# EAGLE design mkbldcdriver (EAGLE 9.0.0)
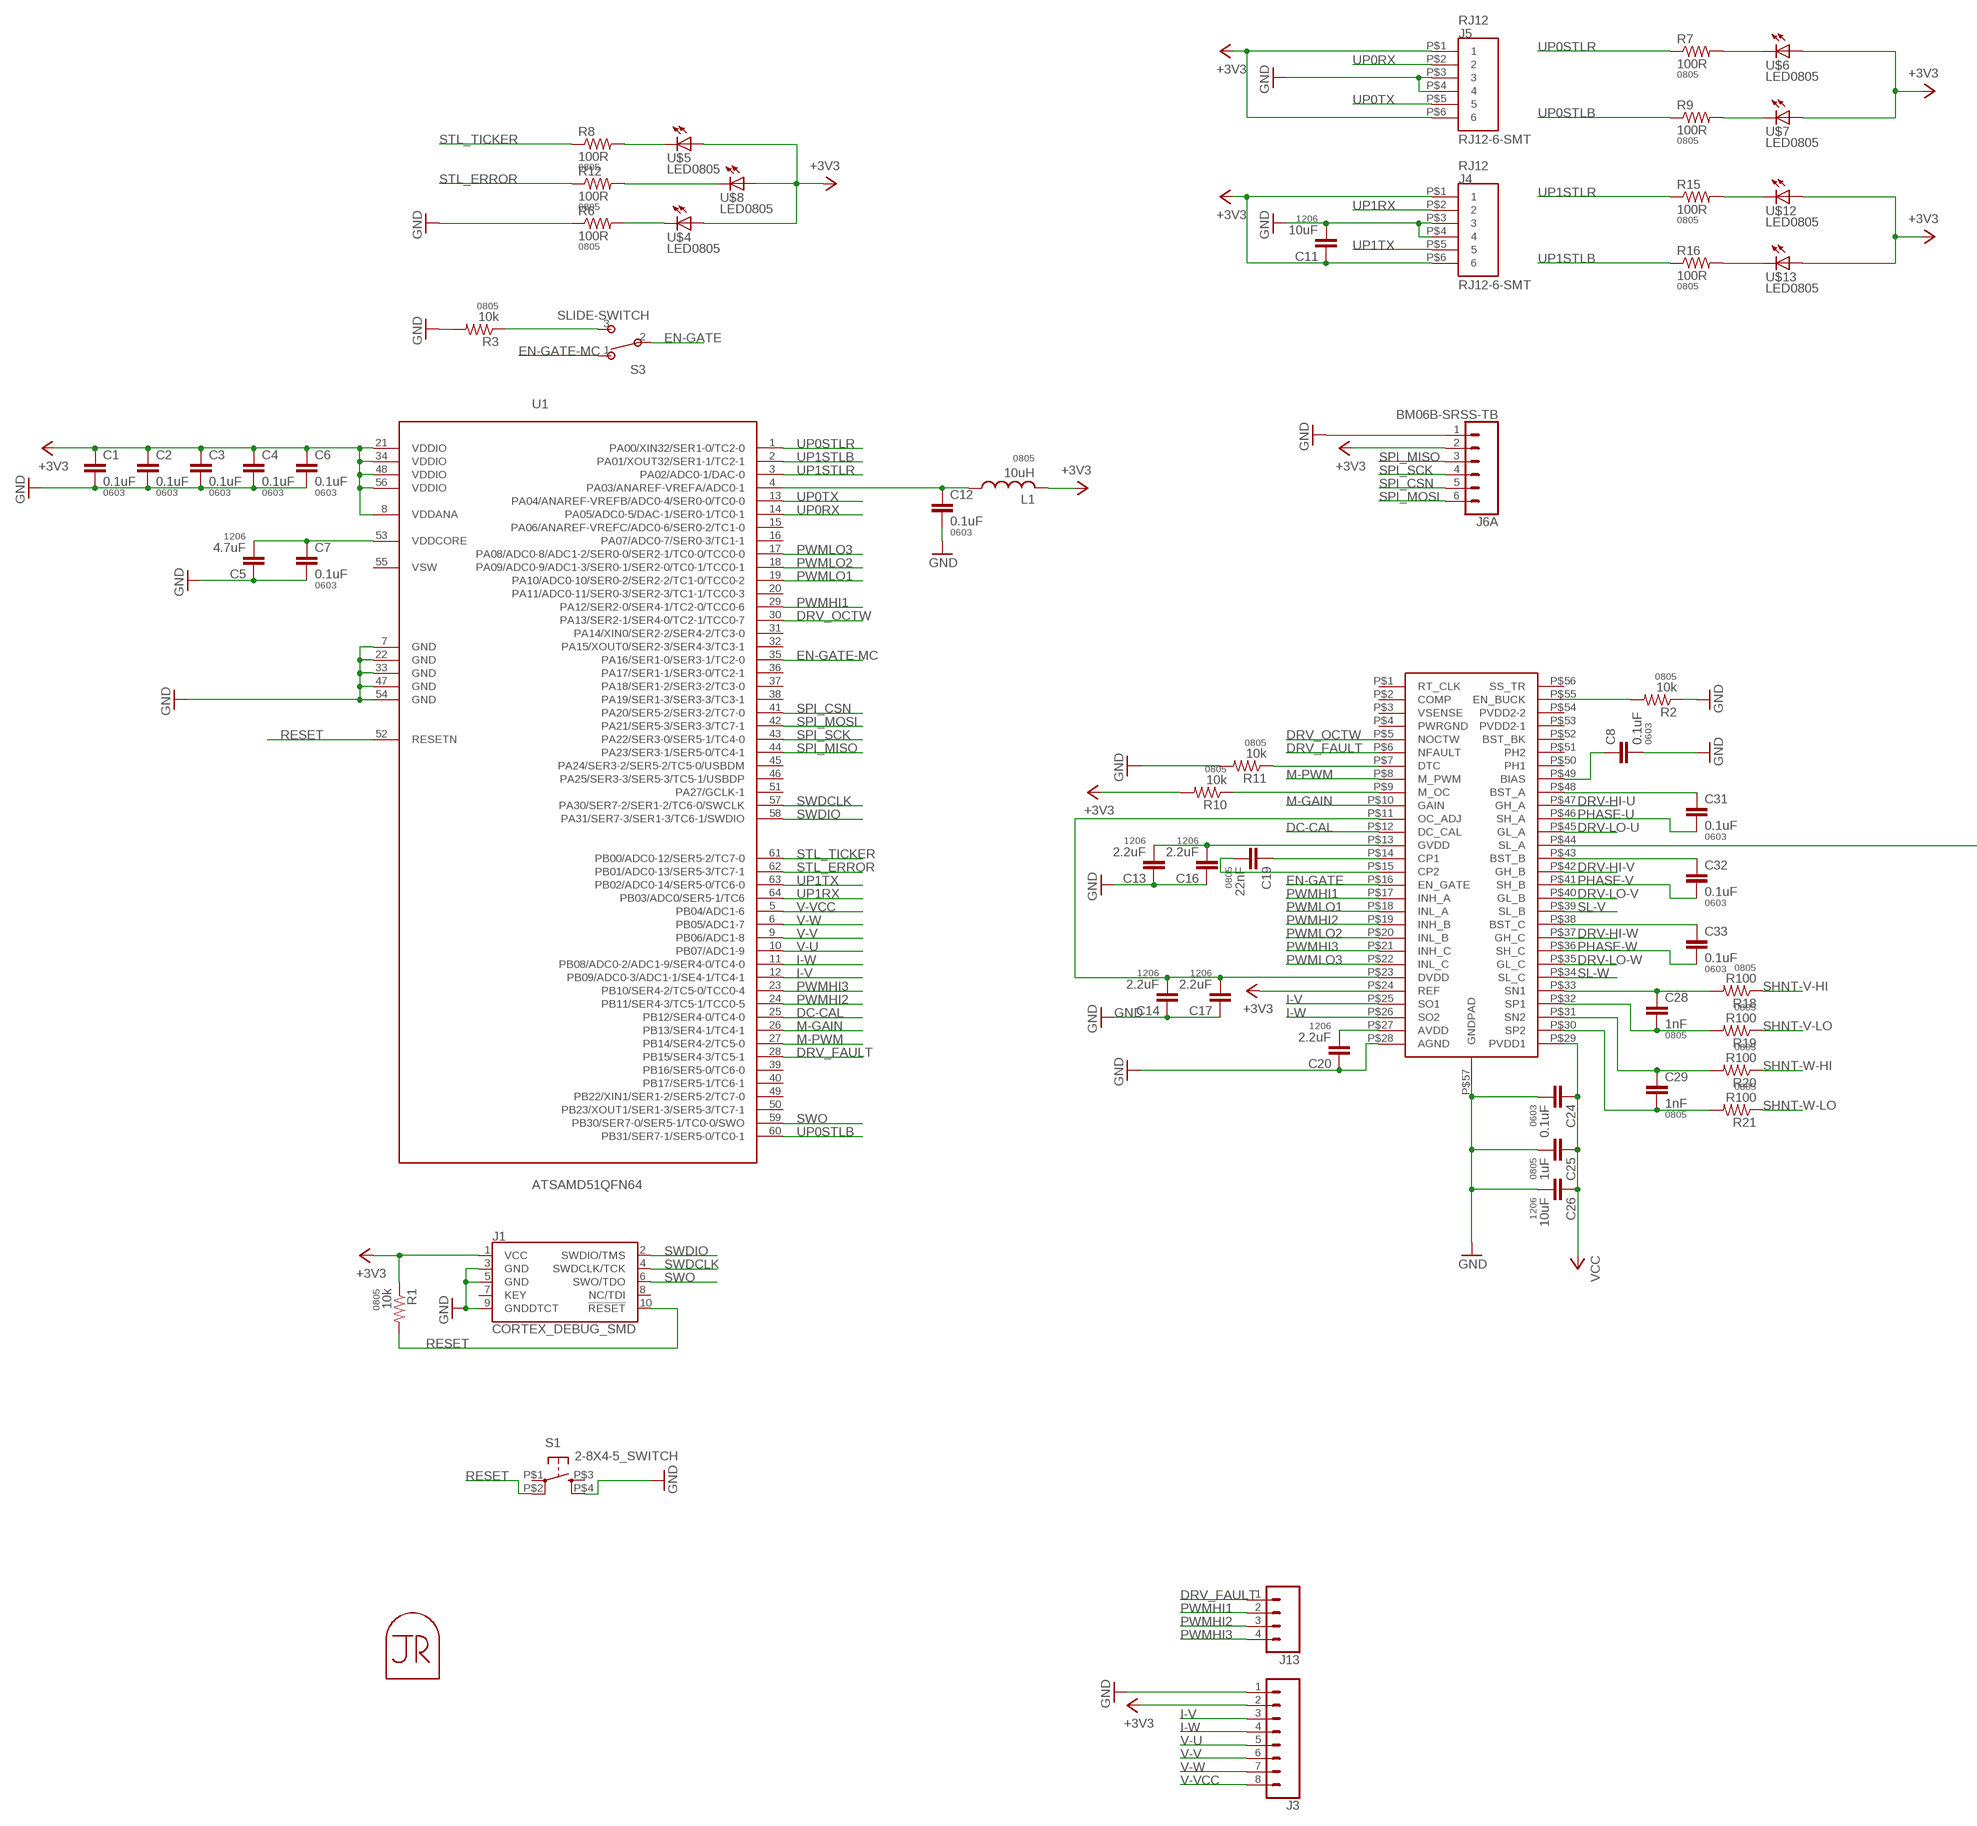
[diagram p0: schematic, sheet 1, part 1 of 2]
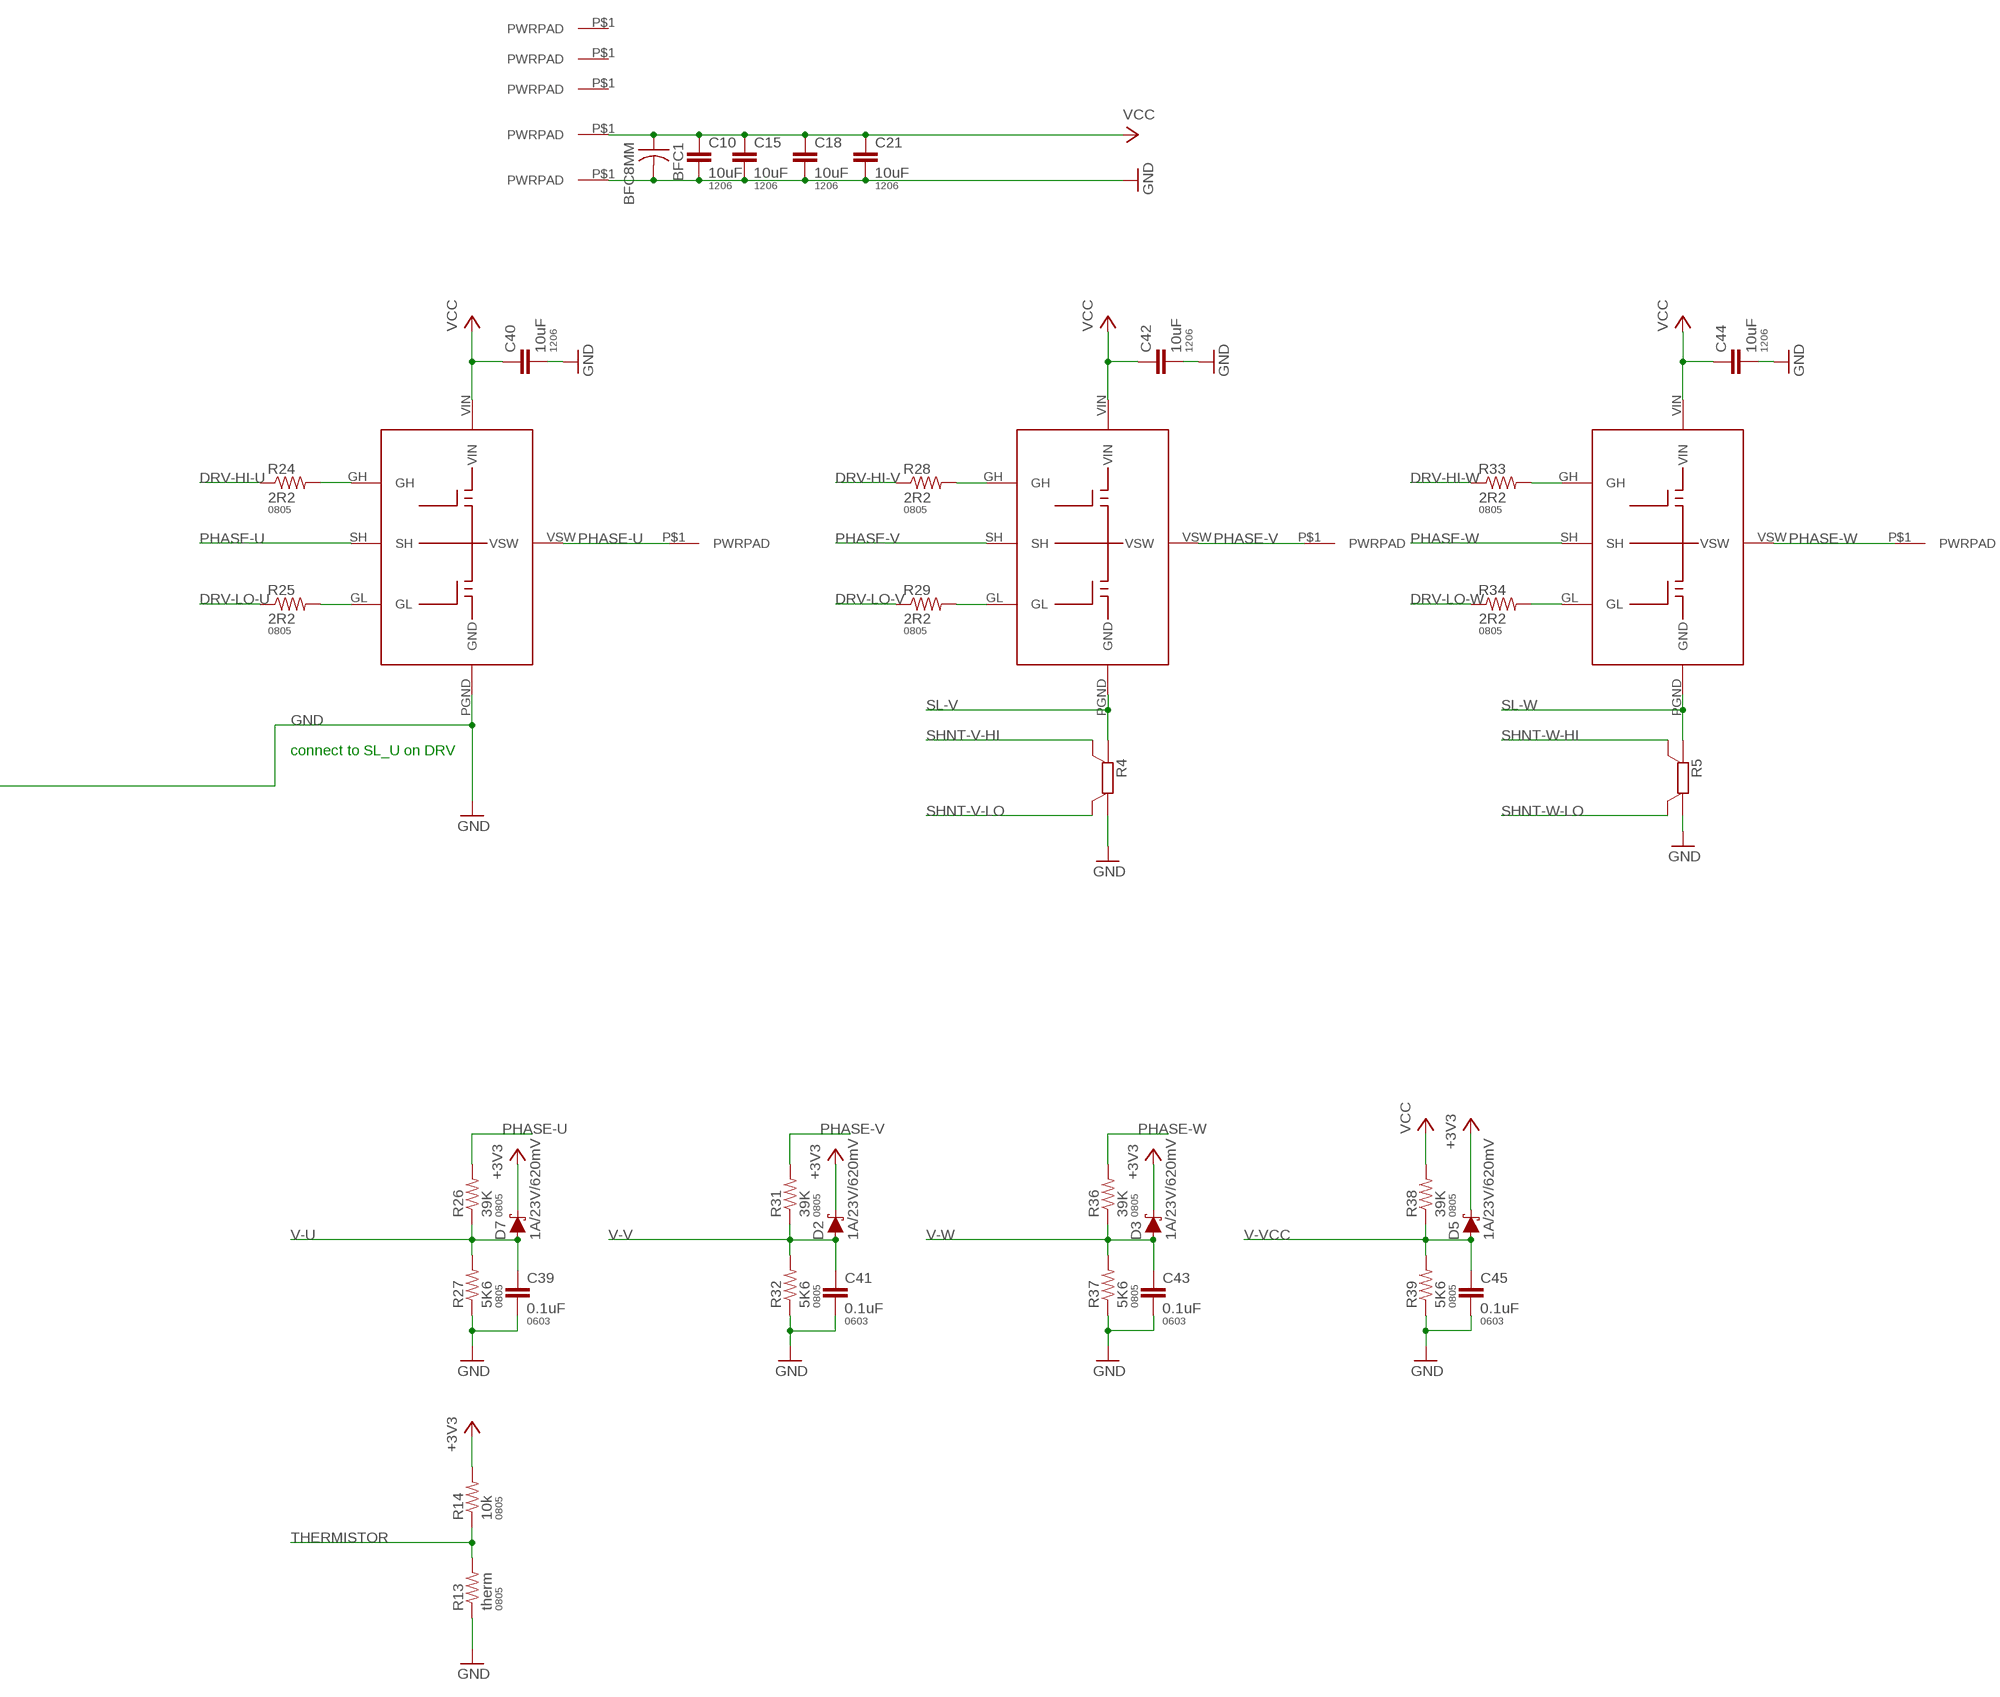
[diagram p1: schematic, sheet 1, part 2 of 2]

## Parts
BFC1  BFC8MM  [BFC-8MM]
C1  0.1uF  CAP0603-CAP  [0603-CAP]
C2  0.1uF  CAP0603-CAP  [0603-CAP]
C3  0.1uF  CAP0603-CAP  [0603-CAP]
C4  0.1uF  CAP0603-CAP  [0603-CAP]
C5  4.7uF  CAP1206  [1206]
C6  0.1uF  CAP0603-CAP  [0603-CAP]
C7  0.1uF  CAP0603-CAP  [0603-CAP]
C8  0.1uF  CAP0603-CAP  [0603-CAP]
C10  10uF  CAP1206  [1206]
C11  10uF  CAP1206  [1206]
C12  0.1uF  CAP0603-CAP  [0603-CAP]
C13  2.2uF  CAP1206  [1206]
C14  2.2uF  CAP1206  [1206]
C15  10uF  CAP1206  [1206]
C16  2.2uF  CAP1206  [1206]
C17  2.2uF  CAP1206  [1206]
C18  10uF  CAP1206  [1206]
C19  22nF  CAP0805  [0805]
C20  2.2uF  CAP1206  [1206]
C21  10uF  CAP1206  [1206]
C24  0.1uF  CAP0603-CAP  [0603-CAP]
C25  1uF  CAP0805  [0805]
C26  10uF  CAP1206  [1206]
C28  1nF  CAP0805  [0805]
C29  1nF  CAP0805  [0805]
C31  0.1uF  CAP0603-CAP  [0603-CAP]
C32  0.1uF  CAP0603-CAP  [0603-CAP]
C33  0.1uF  CAP0603-CAP  [0603-CAP]
C39  0.1uF  CAP0603-CAP  [0603-CAP]
C40  10uF  CAP1206  [1206]
C41  0.1uF  CAP0603-CAP  [0603-CAP]
C42  10uF  CAP1206  [1206]
C43  0.1uF  CAP0603-CAP  [0603-CAP]
C44  10uF  CAP1206  [1206]
C45  0.1uF  CAP0603-CAP  [0603-CAP]
D2  1A/23V/620mV  DIODE-SCHOTTKY-BAT20J  [SOD-323]
D3  1A/23V/620mV  DIODE-SCHOTTKY-BAT20J  [SOD-323]
D5  1A/23V/620mV  DIODE-SCHOTTKY-BAT20J  [SOD-323]
D7  1A/23V/620mV  DIODE-SCHOTTKY-BAT20J  [SOD-323]
J1  CORTEX_DEBUG_SMD  [SAMTECH_FTSH-105-01]
J3  CONN_08NO_SILK_FEMALE_PTH  [1X08_NO_SILK]
J4  RJ12-6-SMT  [RJ12-6-SMT]
J5  RJ12-6-SMT  [RJ12-6-SMT]
J6  BM06B-SRSS-TB  JST_6_PIN_HORIZONTAL  [JST-6-SMD-HORI-1.0MM]
J7  PWRPAD  [PWRPAD_M3-PEM-MOUNT]
J8  PWRPAD  [PWRPAD_M3-PEM-MOUNT]
J9  PWRPAD  [PWRPAD_M3-PEM-MOUNT]
J10  PWRPAD  [PWRPAD_M3-PEM-MOUNT]
J11  PWRPAD  [PWRPAD_M3-PEM-MOUNT]
J12  PWRPADM3  [PWRPAD_3-25MM]
J13  CONN_041X04_NO_SILK  [1X04_NO_SILK]
J14  PWRPADM3  [PWRPAD_3-25MM]
J15  PWRPADM3  [PWRPAD_3-25MM]
L1  10uH  INDUCTOR-0805  [0805]
R1  10k  RESISTOR0805-RES  [0805]
R2  10k  RESISTOR0805-RES  [0805]
R3  10k  RESISTOR0805-RES  [0805]
R4  R_SHUNT2512  [R2512]
R5  R_SHUNT2512  [R2512]
R6  100R  RESISTOR0805-RES  [0805]
R7  100R  RESISTOR0805-RES  [0805]
R8  100R  RESISTOR0805-RES  [0805]
R9  100R  RESISTOR0805-RES  [0805]
R10  10k  RESISTOR0805-RES  [0805]
R11  10k  RESISTOR0805-RES  [0805]
R12  100R  RESISTOR0805-RES  [0805]
R13  therm  RESISTOR0805-RES  [0805]
R14  10k  RESISTOR0805-RES  [0805]
R15  100R  RESISTOR0805-RES  [0805]
R16  100R  RESISTOR0805-RES  [0805]
R18  R100  RESISTOR0805-RES  [0805]
R19  R100  RESISTOR0805-RES  [0805]
R20  R100  RESISTOR0805-RES  [0805]
R21  R100  RESISTOR0805-RES  [0805]
R24  2R2  RESISTOR0805-RES  [0805]
R25  2R2  RESISTOR0805-RES  [0805]
R26  39K  RESISTOR0805-RES  [0805]
R27  5K6  RESISTOR0805-RES  [0805]
R28  2R2  RESISTOR0805-RES  [0805]
R29  2R2  RESISTOR0805-RES  [0805]
R31  39K  RESISTOR0805-RES  [0805]
R32  5K6  RESISTOR0805-RES  [0805]
R33  2R2  RESISTOR0805-RES  [0805]
R34  2R2  RESISTOR0805-RES  [0805]
R36  39K  RESISTOR0805-RES  [0805]
R37  5K6  RESISTOR0805-RES  [0805]
R38  39K  RESISTOR0805-RES  [0805]
R39  5K6  RESISTOR0805-RES  [0805]
S1  2-8X4-5_SWITCH  [TACT-SWITCH-KMR6]
S3  SLIDE-SWITCH  [AYZ0102AGRLC]
U1  ATSAMD51QFN64  [QFN-64-9X9MM]
U2  DRV8302  [HTSSOP-56]
U$4  LED0805  [LED0805]
U$5  LED0805  [LED0805]
U$6  LED0805  [LED0805]
U$7  LED0805  [LED0805]
U$8  LED0805  [LED0805]
U$9  INTEGRATED_HALF-CSD88599SON  [SON-5X6]
U$10  INTEGRATED_HALF-CSD88599SON  [SON-5X6]
U$11  INTEGRATED_HALF-CSD88599SON  [SON-5X6]
U$12  LED0805  [LED0805]
U$13  LED0805  [LED0805]
U$14  JRTOMBSTONE  [JRTOMBSTONE]

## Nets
+3V3: C1.1 C2.1 C3.1 C4.1 C6.1 C11.1 D2.C D3.C D5.C D7.C J1.1(VCC) J3.2 J4.P$1 J4.P$6 J5.P$1 J5.P$6 J6.2 L1.2 R1.1 R10.2 R14.2 U1.8(VDDANA) U1.21(VDDIO) U1.34(VDDIO) U1.48(VDDIO) U1.56(VDDIO) U2.P$24(REF) U$4.1(A) U$5.1(A) U$6.1(A) U$7.1(A) U$8.1(A) U$12.1(A) U$13.1(A)
CP1: C19.1 U2.P$14(CP1)
CP2: C19.2 U2.P$15(CP2)
DC-CAL: U1.25(PB12/SER4-0/TC4-0) U2.P$12(DC_CAL)
DRV-HI-U: R24.1 U2.P$47(GH_A)
DRV-HI-V: R28.1 U2.P$42(GH_B)
DRV-HI-W: R33.1 U2.P$37(GH_C)
DRV-LO-U: R25.1 U2.P$45(GL_A)
DRV-LO-V: R29.1 U2.P$40(GL_B)
DRV-LO-W: R34.1 U2.P$35(GL_C)
DRV_FAULT: J13.1 U1.28(PB15/SER4-3/TC5-1) U2.P$6(NFAULT)
DRV_OCTW: U1.30(PA13/SER2-1/SER4-0/TC2-1/TCC0-7) U2.P$5(NOCTW)
EN-GATE: S3.2 U2.P$16(EN_GATE)
EN-GATE-MC: S3.1 U1.35(PA16/SER1-0/SER3-1/TC2-0)
GND: BFC1.P$2 C1.2 C2.2 C3.2 C4.2 C5.1 C6.2 C7.2 C8.2 C10.2 C11.2 C12.2 C13.1 C14.1 C15.2 C16.1 C17.1 C18.2 C20.1 C21.2 C24.2 C25.2 C26.2 C39.2 C40.2 C41.2 C42.2 C43.2 C44.2 C45.2 J1.3(GND) J1.5(GND) J1.9(GNDDTCT) J3.1 J4.P$3 J4.P$4 J5.P$3 J5.P$4 J6.1 J9.P$1(PWRPAD) R2.1 R3.2 R4.A R5.A R6.1 R11.2 R13.1 R27.1 R32.1 R37.1 R39.1 S1.P$4(S1) U1.7(GND) U1.22(GND) U1.33(GND) U1.47(GND) U1.54(GND) U2.P$28(AGND) U2.P$44(SL_A) U2.P$57(GNDPAD) U$9.PGND(GND)
I-V: J3.3 U1.12(PB09/ADC0-3/ADC1-1/SE4-1/TC4-1) U2.P$25(SO1)
I-W: J3.4 U1.11(PB08/ADC0-2/ADC1-9/SER4-0/TC4-0) U2.P$26(SO2)
M-GAIN: U1.26(PB13/SER4-1/TC4-1) U2.P$10(GAIN)
M-PWM: U1.27(PB14/SER4-2/TC5-0) U2.P$8(M_PWM)
N$1: R7.2 U$6.2(C)
N$2: R25.2 U$9.GL
N$3: R24.2 U$9.GH
N$4: R28.2 U$10.GH
N$5: R33.2 U$11.GH
N$6: R34.2 U$11.GL
N$7: C33.1 U2.P$38(BST_C)
N$8: C32.1 U2.P$43(BST_B)
N$9: C31.1 U2.P$48(BST_A)
N$10: R2.2 U2.P$55(EN_BUCK)
N$11: C20.2 U2.P$27(AVDD)
N$13: C28.1 R18.2 U2.P$33(SN1)
N$14: C28.2 R19.2 U2.P$32(SP1)
N$15: C29.1 R20.2 U2.P$31(SN2)
N$16: C29.2 R21.2 U2.P$30(SP2)
N$18: C13.2 C16.2 U2.P$13(GVDD)
N$19: C8.1 U2.P$49(BIAS)
N$20: C14.2 C17.2 U2.P$11(OC_ADJ) U2.P$23(DVDD)
N$21: R11.1 U2.P$7(DTC)
N$22: R9.2 U$7.2(C)
N$23: R12.2 U$8.2(C)
N$24: R29.2 U$10.GL
N$25: R10.1 U2.P$9(M_OC)
N$26: R3.1 S3.3
N$27: R15.2 U$12.2(C)
N$28: R16.2 U$13.2(C)
N$34: C12.1 L1.1 U1.4(PA03/ANAREF-VREFA/ADC0-1)
N$35: R6.2 U$4.2(C)
N$36: R8.2 U$5.2(C)
PHASE-U: C31.2 J7.P$1(PWRPAD) R26.2 U2.P$46(SH_A) U$9.SH U$9.VSW
PHASE-V: C32.2 J10.P$1(PWRPAD) R31.2 U2.P$41(SH_B) U$10.SH U$10.VSW
PHASE-W: C33.2 J11.P$1(PWRPAD) R36.2 U2.P$36(SH_C) U$11.SH U$11.VSW
PWMHI1: J13.2 U1.29(PA12/SER2-0/SER4-1/TC2-0/TCC0-6) U2.P$17(INH_A)
PWMHI2: J13.3 U1.24(PB11/SER4-3/TC5-1/TCC0-5) U2.P$19(INH_B)
PWMHI3: J13.4 U1.23(PB10/SER4-2/TC5-0/TCC0-4) U2.P$21(INH_C)
PWMLO1: U1.19(PA10/ADC0-10/SER0-2/SER2-2/TC1-0/TCC0-2) U2.P$18(INL_A)
PWMLO2: U1.18(PA09/ADC0-9/ADC1-3/SER0-1/SER2-0/TC0-1/TCC0-1) U2.P$20(INL_B)
PWMLO3: U1.17(PA08/ADC0-8/ADC1-2/SER0-0/SER2-1/TC0-0/TCC0-0) U2.P$22(INL_C)
RESET: J1.10(!RESET) R1.2 S1.P$2(P1) U1.52(RESETN)
SHNT-V-HI: R4.SB R18.1
SHNT-V-LO: R4.SA R19.1
SHNT-W-HI: R5.SB R20.1
SHNT-W-LO: R5.SA R21.1
SL-V: R4.B U2.P$39(SL_B) U$10.PGND(GND)
SL-W: R5.B U2.P$34(SL_C) U$11.PGND(GND)
SPI_CSN: J6.5 U1.41(PA20/SER5-2/SER3-2/TC7-0)
SPI_MISO: J6.3 U1.44(PA23/SER3-1/SER5-0/TC4-1)
SPI_MOSI: J6.6 U1.42(PA21/SER5-3/SER3-3/TC7-1)
SPI_SCK: J6.4 U1.43(PA22/SER3-0/SER5-1/TC4-0)
STL_ERROR: R12.1 U1.62(PB01/ADC0-13/SER5-3/TC7-1)
STL_TICKER: R8.1 U1.61(PB00/ADC0-12/SER5-2/TC7-0)
SWDCLK: J1.4(SWDCLK/TCK) U1.57(PA30/SER7-2/SER1-2/TC6-0/SWCLK)
SWDIO: J1.2(SWDIO/TMS) U1.58(PA31/SER7-3/SER1-3/TC6-1/SWDIO)
SWO: J1.6(SWO/TDO) U1.59(PB30/SER7-0/SER5-1/TC0-0/SWO)
THERMISTOR: R13.2 R14.1
UP0RX: J5.P$2 U1.14(PA05/ADC0-5/DAC-1/SER0-1/TC0-1)
UP0STLB: R9.1 U1.60(PB31/SER7-1/SER5-0/TC0-1)
UP0STLR: R7.1 U1.1(PA00/XIN32/SER1-0/TC2-0)
UP0TX: J5.P$5 U1.13(PA04/ANAREF-VREFB/ADC0-4/SER0-0/TC0-0)
UP1RX: J4.P$2 U1.64(PB03/ADC0/SER5-1/TC6)
UP1STLB: R16.1 U1.2(PA01/XOUT32/SER1-1/TC2-1)
UP1STLR: R15.1 U1.3(PA02/ADC0-1/DAC-0)
UP1TX: J4.P$5 U1.63(PB02/ADC0-14/SER5-0/TC6-0)
V-U: C39.1 D7.A J3.5 R26.1 R27.2 U1.10(PB07/ADC1-9)
V-V: C41.1 D2.A J3.6 R31.1 R32.2 U1.9(PB06/ADC1-8)
V-VCC: C45.1 D5.A J3.8 R38.1 R39.2 U1.5(PB04/ADC1-6)
V-W: C43.1 D3.A J3.7 R36.1 R37.2 U1.6(PB05/ADC1-7)
VCC: BFC1.P$1 C10.1 C15.1 C18.1 C21.1 C24.1 C25.1 C26.1 C40.1 C42.1 C44.1 J8.P$1(PWRPAD) R38.2 U2.P$29(PVDD1) U$9.VIN U$10.VIN U$11.VIN
VDDCORE: C5.2 C7.1 U1.53(VDDCORE)
Unconnected: J1.7(KEY) J1.8(NC/TDI) J6.M1 J6.M2 J12.P$1(PWRPAD) J14.P$1(PWRPAD) J15.P$1(PWRPAD) S1.P$1(P) S1.P$3(S) U1.15(PA06/ANAREF-VREFC/ADC0-6/SER0-2/TC1-0) U1.16(PA07/ADC0-7/SER0-3/TC1-1) U1.20(PA11/ADC0-11/SER0-3/SER2-3/TC1-1/TCC0-3) U1.31(PA14/XIN0/SER2-2/SER4-2/TC3-0) U1.32(PA15/XOUT0/SER2-3/SER4-3/TC3-1) U1.36(PA17/SER1-1/SER3-0/TC2-1) U1.37(PA18/SER1-2/SER3-2/TC3-0) U1.38(PA19/SER1-3/SER3-3/TC3-1) U1.39(PB16/SER5-0/TC6-0) U1.40(PB17/SER5-1/TC6-1) U1.45(PA24/SER3-2/SER5-2/TC5-0/USBDM) U1.46(PA25/SER3-3/SER5-3/TC5-1/USBDP) U1.49(PB22/XIN1/SER1-2/SER5-2/TC7-0) U1.50(PB23/XOUT1/SER1-3/SER5-3/TC7-1) U1.51(PA27/GCLK-1) U1.55(VSW) U2.P$1(RT_CLK) U2.P$2(COMP) U2.P$3(VSENSE) U2.P$4(PWRGND) U2.P$50(PH1) U2.P$51(PH2) U2.P$52(BST_BK) U2.P$53(PVDD2-1) U2.P$54(PVDD2-2) U2.P$56(SS_TR)

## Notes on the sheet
- connect to SL_U on DRV

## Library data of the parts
BFC1 = power:BFC
C1-C4 C6-C8 C12 C24 C31-C33 C39 C41 C43 C45 = borkedlabs-passives:CAP: Capacitor; PACKAGE: 0603
C5 C10 C11 C13-C18 C20 C21 C26 C40 C42 C44 = borkedlabs-passives:CAP: Capacitor; PACKAGE: 1206
C19 C25 C28 C29 = borkedlabs-passives:CAP: Capacitor; PACKAGE: 0805
D2 D3 D5 D7 = SparkFun-DiscreteSemi:DIODE-SCHOTTKY: Schottky diode; PROD_ID: DIO-11623
J1 = SparkFun-Connectors:CORTEX_DEBUG: Cortex Debug Connector - 10 pin Supports JTAG debug, Serial Wire debug, and Serial Wire Viewer. PTH and SMD connector options available. General Connector Information Products: PTH Connector -via Digi-Key SparkFun PSoc SparkFun T
J3 = SparkFun-Connectors:CONN_08: Multi connection point. Often used as Generic Header-pin footprint for 0.1 inch spaced/style header connections On any of the 0.1 inch spaced packages, you can populate with these: Break Away Headers - Straight (PRT-00116) Break Away Male Headers - Right Angle (PRT-00553) Female Headers (PRT-00115)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; PROD_ID: CONN-08438
J4 J5 = connector:RJ12-6-SMT
J6 = SparkFun-Connectors:JST_6_PIN_HORIZONTAL: JST 6 pin horizontal connector JST-SH type. Here is the connector we sell at SparkFun: name (XXX-00000) Datasheet It was used on these SparkFun products: name (XXX-00000) name (XXX-00000); PROD_ID: XXX-00000
J7-J12 J14 J15 = power:PWRPAD
J13 = SparkFun-Connectors:CONN_04: Multi connection point. Often used as Generic Header-pin footprint for 0.1 inch spaced/style header connections On any of the 0.1 inch spaced packages, you can populate with these: Break Away Headers - Straight (PRT-00116) Break Away Male Headers - Right Angle (PRT-00553) Female Headers (PRT-00115)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; PROD_ID: CONN-09696
L1 = borkedlabs-passives:INDUCTOR; PACKAGE: 0805
R1-R3 R6-R16 R18-R21 R24-R29 R31-R34 R36-R39 = borkedlabs-passives:RESISTOR: Resistor; PACKAGE: 0805
R4 R5 = power:R_SHUNT: Resistor Basic schematic elements and footprints for 0603, 1206, and PTH resistors.
S1 = fab:2-8X4-5_SWITCH
S3 = fab:SLIDE-SWITCH: SMD slide-switch AYZ0102AGRLC as found in the fablab inventory. Includes the mounting holes. Made by Zaerc.
U1 = atsam:ATSAMD51
U2 = power:DRV8302
U$4-U$8 U$12 U$13 = lights:LED: LED
U$9-U$11 = power:INTEGRATED_HALF-CSD88599
U$14 = connector:JRTOMBSTONE

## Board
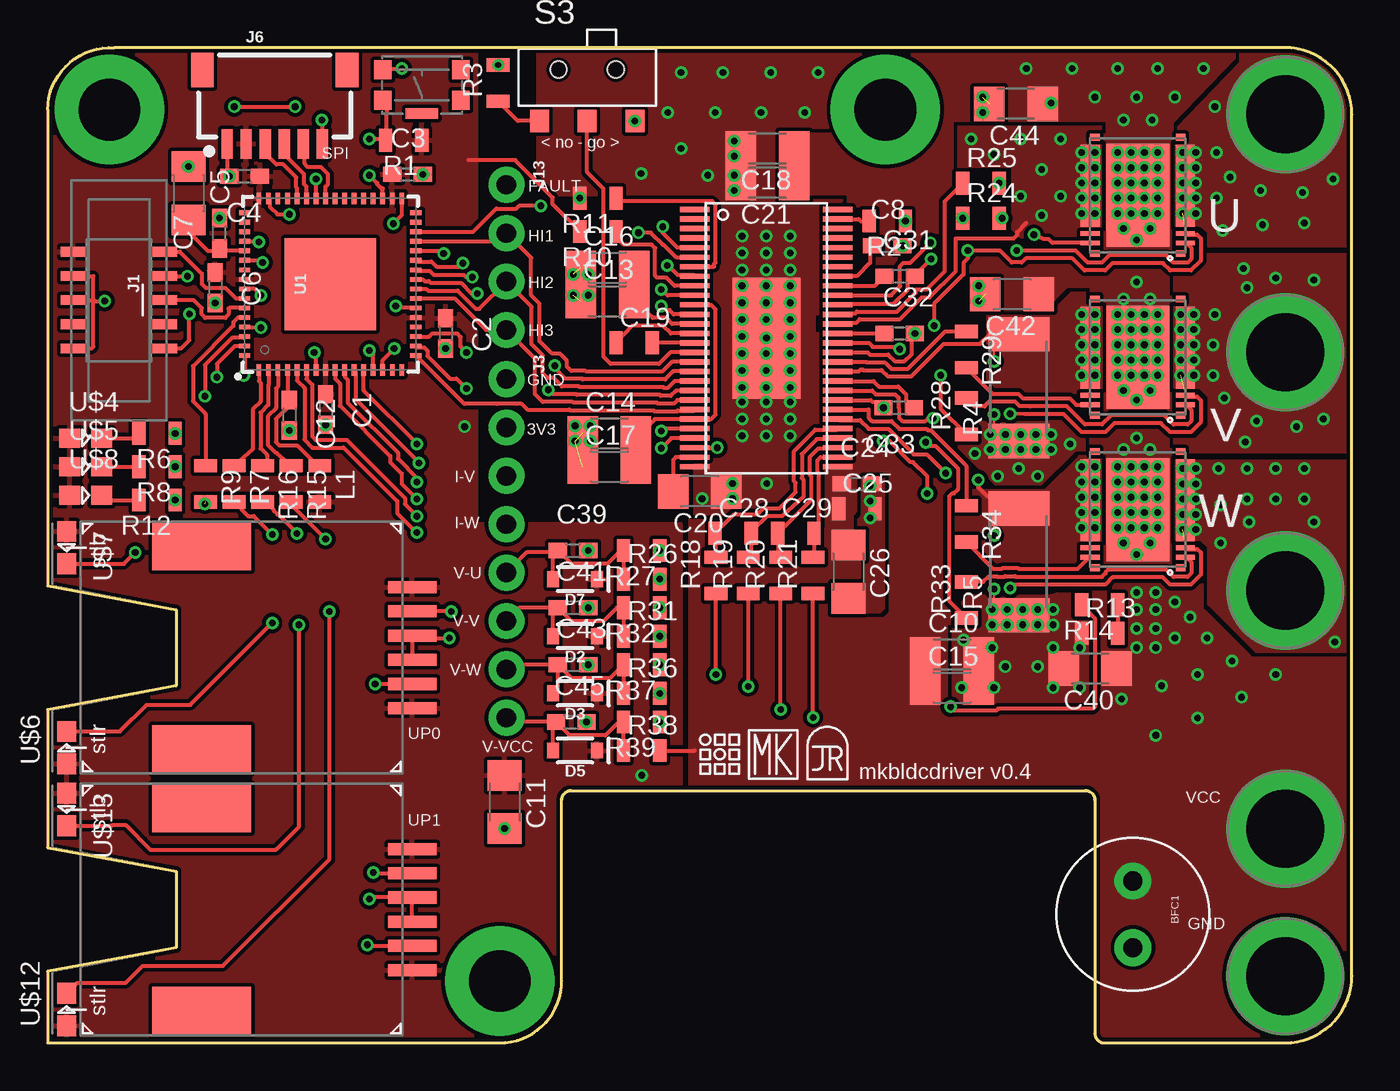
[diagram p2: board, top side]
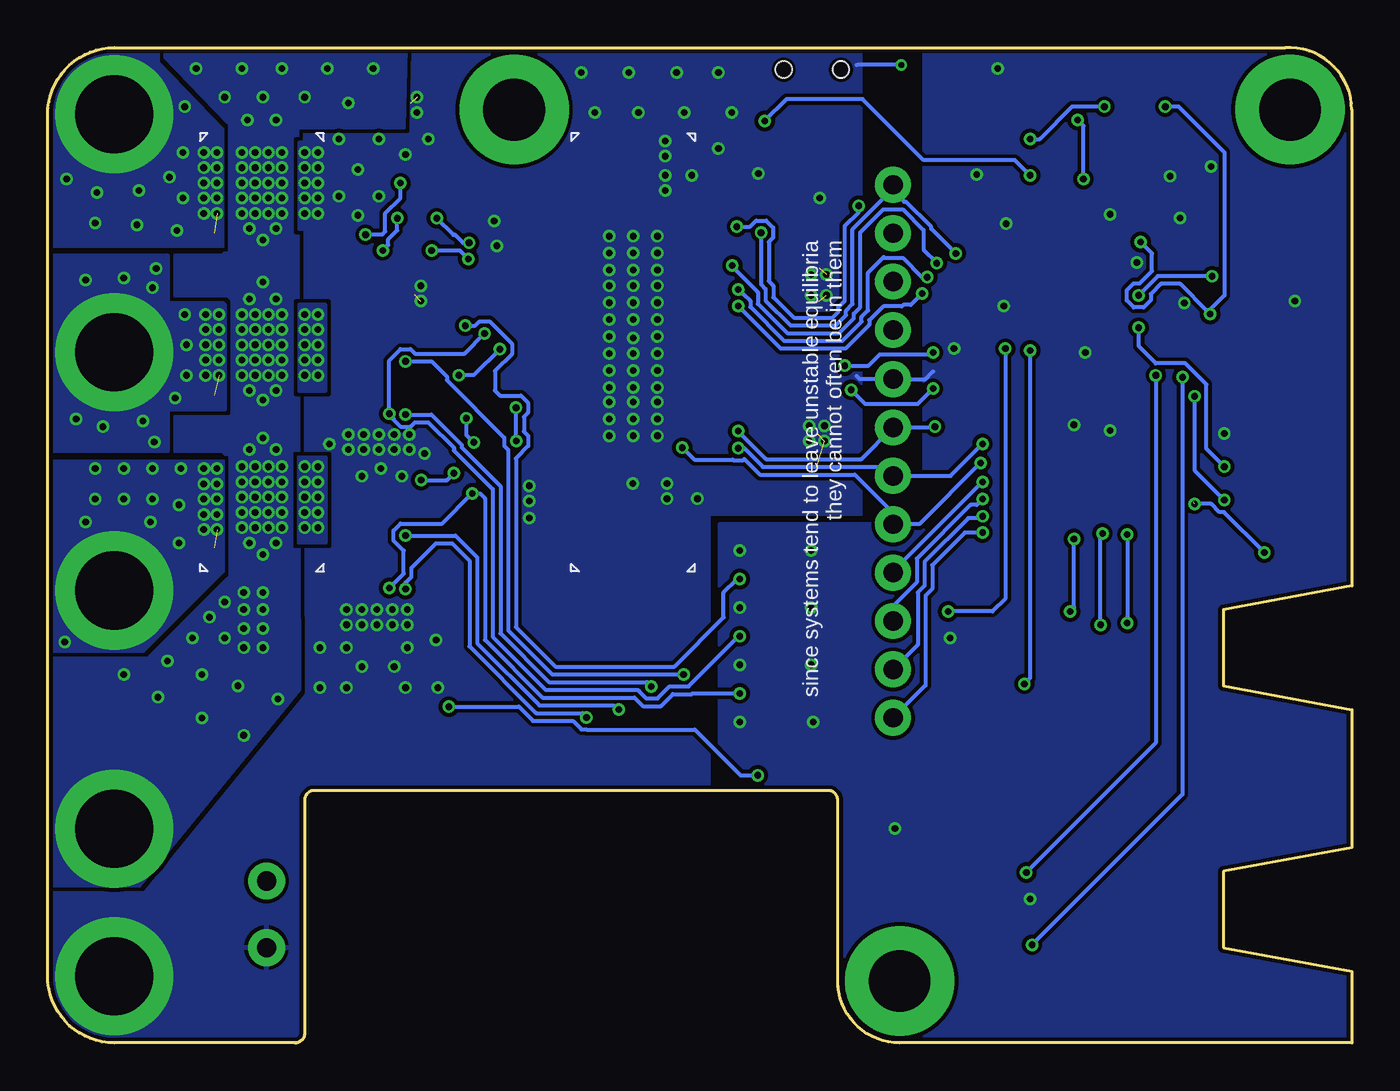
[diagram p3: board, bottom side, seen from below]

Size 68.5 x 52.25 mm. Coordinates in mm from the lower left corner, seen from the top.
Outline: 0,49 arc-92 3.5,52.25 65,52.25 arc-90 68.5,48.75 68.5,3.5 arc-90 65,0 55.5,0 arc-90 55,0.5 55,12.75 arc90 54.5,13.25 27.5,13.25 arc90 27,12.75 27,3.25 arc-90 23.75,0 0,0 0,3.75 6.75,5 6.75,9 0,10.25 0,17.5 6.75,18.75 6.75,22.75 0,24 0,49
Copper layers (1*16): Top 0.035mm / dielectric 1.5mm / Bottom 0.035mm
Design rules "default *": minimum track width 8mil, minimum drill 0.35mm, track to track 8mil, track to pad 8mil, pad to pad 8mil, via to via 8mil, smd to smd 8mil, copper to edge 8mil, drill to drill 8mil, minimum pad ring 10mil, minimum via ring 6mil, stop-mask expansion 4mil, vias tented up to drill 20mil, thermal gap 8mil

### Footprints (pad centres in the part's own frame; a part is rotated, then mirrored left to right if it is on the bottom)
BFC-8MM = drill 1 pad 1.93: P$1 -1.75,0; P$2 1.75,0
0603-CAP = smd 0.96 x 0.8: 1 -0.8,0; 2 0.8,0
1206 = smd 1.6 x 1.8: 1 -1.4,0; 2 1.4,0
0805 = smd 0.7 x 1.2: 1 -0.95,0; 2 0.95,0
SOD-323 = smd 0.63 x 0.83: A 1.15,0; C -1.15,0
SAMTECH_FTSH-105-01 = smd 0.508 x 1.27: 1 -2.54,-2.413; 2 -2.54,2.413; 3 -1.27,-2.413; 4 -1.27,2.413; 5 0,-2.413; 6 0,2.413; 7 1.27,-2.413; 8 1.27,2.413; 9 2.54,-2.413; 10 2.54,2.413
1X08_NO_SILK = drill 1.016 pad 1.88: 1 0,0; 2 2.54,0; 3 5.08,0; 4 7.62,0; 5 10.16,0; 6 12.7,0; 7 15.24,0; 8 17.78,0
RJ12-6-SMT = smd 0.635 x 2.54: P$1 -3.175,17.399; P$2 -1.905,17.399; P$3 -0.635,17.399; P$4 0.635,17.399; P$5 1.905,17.399; P$6 3.175,17.399 | smd 2.54 x 5.207: P$7 -5.334,6.35; P$8 5.334,6.35
JST-6-SMD-HORI-1.0MM = smd 0.6 x 1.55: 1 -2.5,-4.775; 2 -1.5,-4.775; 3 -0.5,-4.775; 4 0.5,-4.775; 5 1.5,-4.775; 6 2.5,-4.775 | smd 1.2 x 1.8: M1 -3.8,-0.9; M2 3.8,-0.9
PWRPAD_M3-PEM-MOUNT = drill 4.1 pad 6.2: P$1 0,0
PWRPAD_3-25MM = drill 3.25 pad 5.75: P$1 0,0
1X04_NO_SILK = drill 1.016 pad 1.88: 1 0,0; 2 2.54,0; 3 5.08,0; 4 7.62,0
R2512 = smd 1.8 x 3.2: A -2.8,0; B 2.8,0 | smd 0.5 x 0.5: SA -1.414,1.3; SB 1.386,1.3
TACT-SWITCH-KMR6 = smd 0.9 x 1: P$1 -2.05,0.8; P$2 2.05,0.8; P$3 -2.05,-0.8; P$4 2.05,-0.8 | smd 1.7 x 0.55: P$5 0,1.5
AYZ0102AGRLC = smd 1 x 1.2: 1 2.5,-2.3; 2 0,-2.3; 3 -2.5,-2.3 | hole 0.85: -1.5,0.4; 1.5,0.4
QFN-64-9X9MM = smd 0.6 x 0.25: 1 -4.5,3.75; 2 -4.5,3.25; 3 -4.5,2.75; 4 -4.5,2.25; 5 -4.5,1.75; 6 -4.5,1.25; 7 -4.5,0.75; 8 -4.5,0.25; 9 -4.5,-0.25; 10 -4.5,-0.75; 11 -4.5,-1.25; 12 -4.5,-1.75; 13 -4.5,-2.25; 14 -4.5,-2.75; 15 -4.5,-3.25; 16 -4.5,-3.75; 33 4.5,-3.75; 34 4.5,-3.25; 35 4.5,-2.75; 36 4.5,-2.25; 37 4.5,-1.75; 38 4.5,-1.25; 39 4.5,-0.75; 40 4.5,-0.25; 41 4.5,0.25; 42 4.5,0.75; 43 4.5,1.25; 44 4.5,1.75; 45 4.5,2.25; 46 4.5,2.75; 47 4.5,3.25; 48 4.5,3.75 | smd 0.25 x 0.6: 17 -3.75,-4.5; 18 -3.25,-4.5; 19 -2.75,-4.5; 20 -2.25,-4.5; 21 -1.75,-4.5; 22 -1.25,-4.5; 23 -0.75,-4.5; 24 -0.25,-4.5; 25 0.25,-4.5; 26 0.75,-4.5; 27 1.25,-4.5; 28 1.75,-4.5; 29 2.25,-4.5; 30 2.75,-4.5; 31 3.25,-4.5; 32 3.75,-4.5; 49 3.75,4.5; 50 3.25,4.5; 51 2.75,4.5; 52 2.25,4.5; 53 1.75,4.5; 54 1.25,4.5; 55 0.75,4.5; 56 0.25,4.5; 57 -0.25,4.5; 58 -0.75,4.5; 59 -1.25,4.5; 60 -1.75,4.5; 61 -2.25,4.5; 62 -2.75,4.5; 63 -3.25,4.5; 64 -3.75,4.5 | smd 4.826 x 4.826: P$1 0,0
HTSSOP-56 = smd 1.549 x 0.279: P$1 -3.75,6.75; P$2 -3.75,6.25; P$3 -3.75,5.75; P$4 -3.75,5.25; P$5 -3.75,4.75; P$6 -3.75,4.25; P$7 -3.75,3.75; P$8 -3.75,3.25; P$9 -3.75,2.75; P$10 -3.75,2.25; P$11 -3.75,1.75; P$12 -3.75,1.25; P$13 -3.75,0.75; P$14 -3.75,0.25; P$15 -3.75,-0.25; P$16 -3.75,-0.75; P$17 -3.75,-1.25; P$18 -3.75,-1.75; P$19 -3.75,-2.25; P$20 -3.75,-2.75; P$21 -3.75,-3.25; P$22 -3.75,-3.75; P$23 -3.75,-4.25; P$24 -3.75,-4.75; P$25 -3.75,-5.25; P$26 -3.75,-5.75; P$27 -3.75,-6.25; P$28 -3.75,-6.75; P$29 3.75,-6.75; P$30 3.75,-6.25; P$31 3.75,-5.75; P$32 3.75,-5.25; P$33 3.75,-4.75; P$34 3.75,-4.25; P$35 3.75,-3.75; P$36 3.75,-3.25; P$37 3.75,-2.75; P$38 3.75,-2.25; P$39 3.75,-1.75; P$40 3.75,-1.25; P$41 3.75,-0.75; P$42 3.75,-0.25; P$43 3.75,0.25; P$44 3.75,0.75; P$45 3.75,1.25; P$46 3.75,1.75; P$47 3.75,2.25; P$48 3.75,2.75; P$49 3.75,3.25; P$50 3.75,3.75; P$51 3.75,4.25; P$52 3.75,4.75; P$53 3.75,5.25; P$54 3.75,5.75; P$55 3.75,6.25; P$56 3.75,6.75 | smd 3.581 x 6.35: P$57 0,0
LED0805 = smd 1.1 x 1: 1 -0.85,0; 2 0.85,0
SON-5X6 = smd 1 x 0.25: GH -2.5,2.5; GL 2.5,2.5; NC 2.5,2; SH -2.5,2 | smd 0.5 x 0.35: M1 -2.25,3.05; M2 2.25,3.05; M3 -2.25,-3.05; M4 2.25,-3.05 | smd 1 x 4.3: PGND 2.5,-0.5; VSW -2.5,-0.5 | smd 3.3 x 5.4: VIN 0,0

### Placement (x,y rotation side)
BFC1  57,6.75 270 top
C1  14.6,33.25 270 top
C2  20.9,37.25 270 top
C3  18.9,45.6 0 top
C4  10.35,45.5 180 top
C5  7.4,44.61 270 top
C6  8.8,39.65 270 top
C7  9.03,42.5 90 top
C8  44.1,41.85 0 top
C10  47.5,20.4 0 top
C11  24,12.65 270 top
C12  12.7,32.95 270 top
C13  29.4,38.95 0 top
C14  29.5,32 0 top
C15  47.5,18.65 0 top
C16  29.4,40.7 0 top
C17  29.5,30.25 0 top
C18  37.8,46.95 180 top
C19  30.8,36.75 0 top
C20  34.25,28.95 180 top
C21  37.8,45.15 180 top
C24  42.5,29.35 0 top
C25  42.5,28.05 0 top
C26  42.06,24.74 270 top
C28  36,26.75 0 top
C29  39.3,26.75 0 top
C31  44.75,40.25 0 top
C32  44.75,37.25 0 top
C33  44.7,33.35 180 top
C39  27.6,25.85 0 top
C40  54.75,19.65 180 top
C41  27.6,22.85 0 top
C42  50.65,39.3 180 top
C43  27.6,19.85 0 top
C44  50.85,49.3 180 top
C45  27.5,16.85 0 top
D2  27.7,21.35 180 top
D3  27.7,18.35 180 top
D5  27.7,15.35 180 top
D7  27.7,24.35 180 top
J1  3.75,39 270 top
J3  24.1,34.85 270 top
J4  1.75,7 270 top
J5  1.75,20.75 270 top
J6  11.93,51.97 0 top
J7  65,48.75 0 top
J8  65,11.25 0 top
J9  65,3.5 0 top
J10  65,36.25 0 top
J11  65,23.75 0 top
J12  44,49 0 top
J13  24.1,45.05 270 top
J14  3.25,49 0 top
J15  23.75,3.25 0 top
L1  14.3,29.35 270 top
R1  18.7,47.4 180 top
R2  44.1,43.15 180 top
R3  23.66,50.39 90 top
R4  51,34.4 90 top
R5  51,25.25 90 top
R6  5.75,32 180 top
R7  9.8,29.35 270 top
R8  5.75,30.25 180 top
R9  8.3,29.35 270 top
R10  28.9,42.6 180 top
R11  28.9,44.35 180 top
R12  5.75,28.5 180 top
R13  55.25,21.5 0 top
R14  55.25,23 180 top
R15  12.8,29.35 270 top
R16  11.3,29.35 270 top
R18  35.1,24.55 90 top
R19  36.8,24.55 90 top
R20  38.5,24.55 90 top
R21  40.2,24.55 90 top
R24  49.02,43.3 0 top
R25  49.02,45.14 0 top
R26  31.2,24.35 0 top
R27  31.2,25.85 180 top
R28  48.25,32.9 90 top
R29  48.25,36.4 270 top
R31  31.2,21.35 0 top
R32  31.2,22.85 180 top
R33  48.25,23.25 90 top
R34  48.25,27.25 270 top
R36  31.2,18.35 0 top
R37  31.2,19.85 180 top
R38  31.2,15.35 0 top
R39  31.2,16.85 180 top
S1  19.66,50.29 180 top
S3  28.34,50.7 0 top
U1  14.85,39.83 90 top
U2  37.75,37 0 top
U$2  [CBA-SILK-LOGO]  35.3,15.15 0 top
U$3  [MK-LOGO-SILK]  38.1,15.15 0 top
U$4  2,31.75 0 top
U$5  2,30.25 0 top
U$6  1,15.5 90 top
U$7  1,26 270 top
U$8  2,28.75 0 top
U$9  57.25,44.5 180 top
U$10  57.25,36 180 top
U$11  57.25,28 180 top
U$12  1,1.75 90 top
U$13  1,12.25 270 top
U$14  41,14.85 0 top

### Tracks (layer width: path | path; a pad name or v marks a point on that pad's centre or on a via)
+3V3  (via drill 0.35)
  Top 0.203: U2.P$24 32.36,32.25 v32.23,32.12 | R14.2 55,22.3 55,17.65 54.9,17.55 49.93,17.55 49.83,17.45 47.64,17.45 v47.43,17.65 | R10.2 26.53,44.02 26.53,44.38 24.56,46.35 22.1,46.35
  Bottom 0.203: v32.23,32.12 30.76,30.65 25.76,30.65 J3.2 21.94,32.31 v21.9,32.35 | v47.43,17.65 43.75,17.65 43.01,16.91 40.91,16.91 40.46,16.46 40.21,16.46 40.2,16.45 34.5,16.45 32.1,14.05 v31.2,14.05
  pour Top: 22.5,52.25 22.5,27.25 33.25,27.25 33.25,0 0,0 0,52.25
CP1
  Top 0.203: U2.P$14 32.73,37.25 32.33,37.66 30.7,37.66 C19.1
CP2
  Top 0.203: U2.P$15 C19.2
DC-CAL  (via drill 0.35)
  Top 0.203: U2.P$12 32.88,38.25 32.66,38.47 32.46,38.47 v32.23,38.69 | U1.25 19.71,40.08 19.8,39.99 20.03,39.99 20.13,39.9 21.7,39.9 22.26,39.34 v22.58,39.34
  Bottom 0.203: v22.58,39.34 23.17,38.75 23.56,38.75 23.63,38.67 24.62,38.67 25.34,37.95 25.34,37.7 26.6,36.45 29.99,36.45 v32.23,38.69
DRV-HI-U  (via drill 0.35)
  Top 0.203: U2.P$47 44.3,39.25 44.77,39.72 44.77,40.78 44.94,40.95 45.31,40.95 v46.36,42.01
  Bottom 0.203: v46.36,42.01 46.68,42.01 47.1,42.42 47.19,42.42 R24.1
  other vias: 48.06,43.3
DRV-HI-V  (via drill 0.35)
  Top 0.203: U2.P$42 43.14,36.75 43.34,36.55 44.62,36.55 v44.75,36.42 | v46.9,35.05 46.9,33.3 R28.1
  Bottom 0.203: v44.75,36.42 46.12,35.05 v46.9,35.05
DRV-HI-W  (via drill 0.35)
  Top 0.203: U2.P$37 43.3,34.25 43.5,34.05 44.51,34.05 44.69,33.88 44.69,33.35 44.72,33.32 44.72,32.82 44.89,32.65 46.11,32.65 46.26,32.8 v46.51,32.8 | v46.12,31.53 46.3,31.35 46.62,31.35 47.8,30.17 47.8,29.05 47.61,28.85 47.52,28.85 47.34,28.68 47.34,23.2 R33.1
  Bottom 0.203: v46.51,32.8 46.51,31.92 v46.12,31.53
DRV-LO-U
  Top 0.203: U2.P$45 41.56,38.3 42.4,38.3 42.5,38.4 44.6,38.4 45.58,39.38 45.58,39.55 46.16,39.55 47.11,40.5 47.11,44.17 48.06,45.13 R25.1
DRV-LO-V
  Top 0.203: U2.P$40 42.99,35.75 43.01,35.73 43.97,35.73 44.32,35.38 45.18,35.38 47.15,37.35 R29.1
DRV-LO-W
  Top 0.203: U2.P$35 | U2.P$35 43.11,33.25 43.11,32.82 43.29,32.65 44.32,32.65 44.72,32.24 46.17,32.24 46.25,32.16 46.38,32.16 48.25,30.3 R34.1
DRV_FAULT  (via drill 0.35)
  Top 0.203: U2.P$6 33,41.25 32.35,41.9 32.31,41.9 31.67,42.54 v31.03,42.54 | U1.28 20.67,41.58 v20.8,41.45
  Bottom 0.203: v31.03,42.54 31.03,39.82 30.79,39.58 30.79,38.97 29.48,37.67 27.1,37.67 26.56,38.21 26.56,38.45 26.22,38.79 26.22,42.73 24.1,44.84 | 24.1,44.84 J13.1 | 24.1,44.84 24.1,44.75 23.51,44.16 23.42,44.16 22.09,42.84 22.09,42.74 v20.8,41.45
DRV_OCTW  (via drill 0.35)
  Top 0.203: U2.P$5 | U2.P$5 33.07,41.75 32.3,42.52 v32.3,42.85 | v25.9,43.95 24.76,43.95 24.62,43.8 23.55,43.8 22.33,42.58 U1.30
  Bottom 0.203: v32.3,42.85 31.61,42.85 31.29,43.17 30.77,43.17 30.4,42.8 30.4,42.27 30.62,42.05 30.62,39.99 30.38,39.74 30.38,39.14 29.31,38.08 27.27,38.08 26.97,38.38 26.97,38.62 26.63,38.96 26.63,42.89 25.9,43.62 v25.9,43.95
EN-GATE
  Top 0.203: U2.P$16 32.71,36.25 32.1,35.64 29.58,35.64 29.2,36.02 29.2,44.85 28.34,45.71 S3.2
EN-GATE-MC  (via drill 0.35)
  Top 0.203: U1.35 17.6,44.85 17.55,44.9 17.49,44.9 17.31,45.07 17.31,45.13 v16.9,45.55
  Bottom 0.203: v16.9,45.55 17.7,46.35 22.5,46.35 25.7,49.55 29.69,49.55 S3.1
  other vias: 30.84,48.4
GND  (via drill 0.3, 0.35)  (6 unrouted)
  Top 0.203: 39.15,37.83 v39.01,37.97 | U1.54 11.19,41.08 v11.3,40.98 | U1.33 18.6,43.46 v18.15,43.01 | U1.22 18.39,38.58 v18.28,38.69 | U1.7 14.1,36.15 v14,36.25 | J6.1 9.43,45.52 C4.2 | S1.P$4 17.66,51.15 v18.6,51.15 | J1.3 1.36,40.25 2.4,40.25 2.4,39.05 | J1.5 2.35,39 2.4,39.05 | J1.9 2.29,36.46 2.3,36.45 2.4,36.55 2.4,39.05 | 2.4,39.05 2.5,38.95 v3,38.95 | U2.P$44 41.56,37.81 42.48,37.81 42.66,37.99 44.77,37.99 45.91,39.14 46.33,39.14 47.7,40.51 47.7,42.24 50.74,42.24 50.92,42.42 50.92,42.57 51.4,43.05 | J5.P$4 J5.P$3 19.28,21.25 v21.1,21.25 | J4.P$4 J4.P$3 16.98,7.64 v16.9,7.55 | U1.47 11.67,44.26 11.67,43.91 12.08,43.5 v12.7,43.5 | 39.15,40.43 v39.01,40.57 | 39.15,31.73 v39.01,31.87
  Bottom 0.203: 26,35 25.85,34.85 J3.1 22.4,34.85 22,35.25 | R3.2 23.67,51.35 26,51.35
  other vias: 36.47,39.75 37.74,39.75 39.01,39.75 36.47,38.86 36.47,37.97 36.47,37.08 36.47,35.31 36.47,36.2 36.47,34.42 37.74,38.86 37.74,37.97 39.01,38.86 39.01,37.08 37.75,37 37.74,36.2 37.74,35.31 37.74,34.42 39.01,36.2 39.01,35.31 39.01,34.42 28.4,40.35 28.4,39.25 20.9,36.45 8.8,38.85 7.4,46.01 9.03,43.3 9.55,45.5 14.6,32.45 12.7,32.15 28.5,32.4 23.66,51.34 19.7,45.6 6.7,32 55,46.75 54.3,46.75 50.3,19.75 48.7,30.95 45.05,43.15 44.9,41.85 48.9,38.95 48.9,39.75 49.1,49.65 49.1,48.85 43.2,29.25 43.2,28.45 43.2,27.55 28.4,22.85 32.15,22.85 32.15,25.85 28.4,25.85 28.4,19.85 28.3,16.85 32.15,16.85 32.15,19.85 24,11.25 27.95,44.35 36.47,42.35 37.74,42.35 39.01,42.35 36.47,41.46 36.47,40.57 37.74,41.46 37.74,40.57 39.01,41.46 36.47,33.65 37.74,33.65 39.01,33.65 36.47,32.76 36.47,31.87 37.74,32.76 37.74,31.87 39.01,32.76 36.07,44.75 36.07,45.55 36.07,46.55 36.07,47.35 39.77,48.85 40.47,50.95 37.97,50.95 37.47,48.85 35.47,50.95 35.07,48.85 33.27,50.95 32.57,48.85 33.27,46.95 31.17,45.65 34.67,45.55 35.97,29.37 35.97,28.57 37.77,29.37 34.37,28.57 55,45.95 54.3,45.95 55,45.15 54.3,45.15 55,44.35 54.3,44.35 55,43.55 54.3,43.55 53.2,47.45 51.1,47.45 48.5,47.45 49.7,46.65 52.2,45.85 51.1,44.45 53.2,44.45 52.2,43.45 51.1,31.95 51.9,31.95 52.7,31.95 50.3,31.95 49.5,31.95 49.5,31.15 50.3,31.15 51.1,31.15 51.9,31.15 52.7,31.15 49.9,29.75 52,29.75 53.7,31.45 51,30.15 49.6,22.75 50.4,22.75 51.2,22.75 52,22.75 52.8,22.75 52,21.95 52.8,21.95 51.2,21.95 50.4,21.95 49.6,21.95 48.1,21.15 48,18.65 49.7,18.65 49.6,20.75 52.8,20.75 52.8,18.65 54.2,18.65 54.2,20.75 52,19.75 27.7,32.4 28.5,31.6 27.7,31.6 27.6,39.25 27.6,40.35
  pour Top (no thermals): 40.5,27.75 34,27.75 34,44 33.5,44.5 25.75,44.5 25.75,52.25 43.25,52.25 43.3,48.05 38.5,48.05 38.55,44.25 41.75,44.25 41.5,44 41.5,38.25 40.25,38.25 40.25,37.25 40.5,37.25
  pour Bottom (rank 6): 54.5,13.25 33.75,13.25 33.75,27.75 25.75,27.75 25.75,52.25 68.5,52.25 68.5,0 55,0 55,12.75
  pour Bottom: 22.5,52.25 22.5,27.25 33.25,27.25 33.25,0 0,0 0,52.25
  pour Top (no thermals): 55.3,41.95 55.3,48.05 47.85,48.05 47.85,46.05 50.7,46.05 50.7,42.75 51.5,41.95
  pour Top (rank 2, no thermals): 49.4,32.55 52.6,32.55 52.8,32.75 53.3,32.75 54.4,31.65 54.4,30.95 54.2,30.95 54,30.75 52.5,29.25 50,29.25 49.9,29.25 47.8,31.35 47.8,32.25 48.1,32.55
  pour Top (no thermals): 48.4,23.45 52.7,23.45 53,23.55 55,23.55 55,17.65 47.6,17.65 47.6,22.65
  pour Bottom (rank 3, no thermals): 53.9,47.25 55.3,47.25 55.3,42.75 53.9,42.75
  pour Top (rank 3, no thermals): 42.8,29.55 42.8,27.65 42.6,27.45 42.6,26.75 43,26.75 43,24.15 42.9,24.05 41.3,24.05 41.3,22.65 43.7,22.65 43.9,22.85 43.9,29.55
I-V  (via drill 0.35)
  Top 0.203: U2.P$25 32.76,31.75 v32.23,31.22 | v19.4,31.45 16.6,34.25 U1.12
  Bottom 0.203: v32.23,31.22 31.91,31.22 30.93,30.24 24.57,30.24 J3.3 21.08,29.77 v19.4,31.45
I-W  (via drill 0.35)
  Top 0.203: U2.P$26 v35.17,31.25 | v35.17,31.25 | U1.11 16.17,35.26 16.17,33.78 v19.5,30.46 v19.5,30.45
  Bottom 0.203: v35.17,31.25 34.53,30.62 32.52,30.62 32.49,30.59 31.96,30.59 31.91,30.64 31.1,29.84 26.1,29.84 24.1,27.84 J3.4 22.72,27.23 v19.5,30.45
M-GAIN  (via drill 0.35)
  Top 0.203: U2.P$10 32.57,39.25 32.49,39.33 32.46,39.33 v32.23,39.55 | v22.3,40.2 21.98,40.2 21.87,40.3 20.3,40.3 20.09,40.51 19.42,40.51 U1.26
  Bottom 0.203: v32.23,39.55 32,39.33 31.97,39.33 31.6,38.95 31.6,38.64 29.82,36.86 26.77,36.86 25.75,37.87 25.75,38.11 25.41,38.46 25.41,40.44 24.6,41.25 24.56,41.22 23.58,41.22 22.57,40.2 v22.3,40.2
M-PWM  (via drill 0.35)
  Top 0.203: v21.8,40.94 21.62,40.75 20.42,40.75 20.16,41.01 19.42,41.01 U1.27 | U2.P$8 33.94,40.3 33.1,40.3 32.59,40.82 v32.54,40.82
  Bottom 0.203: v21.8,40.94 v21.8,40.95 22.5,41.65 22.5,42.67 23.58,43.76 24.62,43.76 25.81,42.56 25.81,38.63 26.16,38.28 26.16,38.04 26.94,37.26 29.65,37.26 31.19,38.8 31.19,39.41 32.54,40.75 v32.54,40.82
N$1  (via drill 0.35)
  Top 0.203: U$6.2 3.8,16.35 5.2,17.75 7.5,17.75 v11.8,22.05 | R7.2 10.54,27.66 10.83,27.66 v11.8,26.69
  Bottom 0.203: v11.8,26.69 v11.8,22.05
N$2  (via drill 0.35)
  Top 0.203: v51.8,42.43 52.33,42.2 52.58,42.2 52.78,42 U$9.GL
  Bottom 0.203: v51.8,42.43 51.78,42.45 50.92,42.45 50.77,42.6 50.77,43.56 49.97,44.36 R25.2
  other vias: 49.97,45.14
N$3  (via drill 0.35)
  Top 0.203: v50.13,43.3 R24.2 | U$9.GH 59.82,41.93 59.88,41.93 60.06,41.75 60.06,41.15 59.88,40.97 59.12,40.97 58.74,41.35 55.76,41.35 55.38,40.97 54.62,40.97 54,41.59 50.92,41.59 v50.9,41.61
  Bottom 0.203: v50.13,43.3 50.13,42.66 50.61,42.18 50.61,41.9 v50.9,41.61
N$4
  Top 0.203: U$10.GH 59.82,33.43 59.88,33.43 60.06,33.25 60.06,32.65 59.88,32.47 59.12,32.47 58.64,32.95 55.86,32.95 55.38,32.47 54.48,32.47 53.53,33.42 51.6,33.42 51.05,33.43 50.82,33.66 49.45,33.66 49.2,33.42 48.68,33.42 R28.2
N$5
  Top 0.203: U$11.GH 59.82,25.43 59.88,25.43 60.06,25.25 60.06,24.65 59.88,24.47 59.12,24.47 58.74,24.85 55.7,24.85 55.56,24.7 55.56,24.65 55.38,24.47 50.86,24.47 50.82,24.51 50.3,24.51 50.25,24.47 49.92,24.47 | 49.92,24.47 | R33.2 49.13,24.2 49.4,24.47 49.92,24.47
N$6
  Top 0.203: U$11.GL 54.68,25.43 54.62,25.43 54.07,24.88 51.03,24.88 50.99,24.92 50.13,24.92 50.08,24.88 49.67,24.88 R34.2
N$7
  Top 0.203: U2.P$38 43.38,34.75 43.66,34.46 44.67,34.46 45.09,34.05 45.09,33.76 C33.1
N$8
  Top 0.203: U2.P$43 C32.1 | C32.1
N$9
  Top 0.203: U2.P$48 43.45,39.75 C31.1
N$10
  Top 0.203: U2.P$55 | U2.P$55 42.6,43.25 42.7,43.15 R2.2
N$11
  Top 0.203: U2.P$27 | U2.P$27 33,30.75 32.85,30.6 C20.2
N$13
  Top 0.203: U2.P$33 41.45,32.2 40.32,32.2 39.2,31.08 39.2,29.48 39.28,29.4 39.28,28.91 38.51,28.14 38.42,28.06 37.61,28.06 37.29,27.74 36.05,27.74 C28.1 35.1,26.7 R18.2
N$14
  Top 0.203: U2.P$32 41.44,31.7 40.39,31.7 39.61,30.91 39.61,29.65 39.69,29.57 39.69,28.66 38.58,27.66 37.77,27.66 36.97,26.85 C28.2 36.95,25.65 R19.2
N$15
  Top 0.203: U2.P$31 41.44,31.2 40.47,31.2 40.01,30.74 40.01,29.82 40.09,29.74 40.09,28.49 C29.1 38.35,25.65 R20.2
N$16
  Top 0.203: U2.P$30 40.6,30.75 40.42,30.57 40.42,29.98 40.5,29.91 40.5,27.1 C29.2 40.25,25.55 R21.2
N$18
  Top 0.203: C16.2 C13.2 31.79,38.06 32.5,38.06 32.81,37.75 U2.P$13
N$19
  Top 0.203: U2.P$49 42.5,40.25 43.2,40.95 43.2,41.75 C8.1
N$20
  Top 0.203: U2.P$11 34.84,38.75 35.08,38.52 35.08,32.98 34.84,32.75 U2.P$23 31.9,32.75 30.9,31.75 | C17.2 30.9,31.75 | 30.9,31.75 C14.2
N$21
  Top 0.203: U2.P$7 | R11.1 30.11,44.19 34.9,44.19 35.08,44.02 35.08,40.98 35,40.91 35,40.75 U2.P$7
N$22  (via drill 0.35)  (1 unrouted)
  Top 0.203: U$7.2 4,25.15 v4.6,25.75
  Bottom 0.203: v4.6,25.75 6.72,27.87 6.96,27.87 7.39,28.3 v8.27,28.3
N$23
  Top 0.203: U$8.2 3.1,28.5 R12.2
N$24
  Top 0.203: U$10.GL 54.03,33.5 53.69,33.83 51.22,33.83 50.99,34.07 49.63,34.07 R29.2
N$25
  Top 0.203: U2.P$9 32.93,39.75 32.49,40.18 32,40.18 31.91,40.28 31.91,41.73 31.73,41.91 30.25,41.91 29.85,42.3 R10.1
N$26
  Top 0.203: S3.3 24.69,48.4 R3.1
N$27  (via drill 0.35)
  Top 0.203: U$12.2 1.55,3.15 4.1,3.15 5,4.05 9.2,4.05 14.8,9.65 v14.8,22.65 | v14.6,26.45 12.8,28.25 R15.2
  Bottom 0.203: v14.8,22.65 14.6,22.85 v14.6,26.45
N$28  (via drill 0.35)
  Top 0.203: U$13.2 3.35,11.4 3.4,11.45 4.1,11.45 5.4,10.15 12,10.15 13.2,11.35 v13.2,21.95 | R16.2 11.45,28.4 11.9,27.95 11.9,27.92 12.07,27.74 12.1,27.74 v13.1,26.75
  Bottom 0.203: v13.2,21.95 13.2,26.65 v13.1,26.75
N$34
  Top 0.203: U1.4 12.6,34.06 C12.1 | C12.1 12.5,33.76 | L1.1 14.18,30.29 13.1,31.37 12.17,31.37 11.99,31.54 11.99,32.76 12.7,33.46 C12.1
N$35
  Top 0.203: U$4.2 4.55,31.75 R6.2
N$36
  Top 0.203: U$5.2 R8.2
PHASE-U  (via drill 0.35)  (1 unrouted)
  Top 0.203: U2.P$46 41.56,38.8 44.43,38.8 45.17,39.55 45.17,39.87 C31.2 45.55,40.3 v46.4,41.15 | U$9.SH 59.82,42.43 60.38,42.43 60.56,42.25 60.56,41.07 60.05,40.56 58.95,40.56 58.58,40.94 55.92,40.94 55.55,40.56 54.45,40.56 53.83,41.19 51.37,41.19 51.16,40.98 50.64,40.98 50.03,41.58 48.36,41.58 v48.33,41.61 48.33,41.18 48.11,40.96 48.11,40.35 46.56,38.8 v46.56,37.66
  Bottom 0.203: v48.33,41.61 46.86,41.61 v46.4,41.15 | v46.56,37.66 46.04,37.66 45.81,37.88 45.29,37.88 44.12,36.71 44.12,36.16 45,35.28 45,34.25 44.73,33.98 43.64,33.98 43.27,33.61 43.27,33.09 43.48,32.87 43.48,32.09 43.26,31.87 43.26,31.34 43.91,30.7 43.91,21.83 41.83,19.76 35.59,19.76 33,22.34 33,23.65 32.3,24.35 R26.2
  other vias: 59.6,46.75 32.15,24.35 60.3,46.75 59.6,45.95 60.3,45.95 59.6,45.15 60.3,45.15 59.6,44.35 60.3,44.35 59.6,43.55 60.3,43.55 61.4,46.75 62.1,45.45 63.7,44.75 65.9,44.65 67.5,45.35 61.3,49.15 61.4,44.35 61.7,42.65 63.8,42.95 66,43.05
  pour Top (rank 3, no thermals): 59.3,42.95 59.3,47.95 62.7,51.45 62.7,52.25 68.5,52.25 68.5,41.85 61,41.85 61,42.55 60.5,42.95
  pour Bottom (rank 3, no thermals): 59.3,41.85 59.3,47.95 62.7,51.45 62.7,52.25 68.5,52.25 68.5,41.85
PHASE-V  (via drill 0.35)  (1 unrouted)
  Top 0.203: U2.P$41 43.06,36.25 43.17,36.14 44.14,36.14 44.49,35.79 45.01,35.79 45.38,36.16 45.38,37.08 C32.2 | U$10.SH 59.82,33.93 60.38,33.93 60.56,33.75 60.56,32.57 60.05,32.06 58.95,32.06 58.48,32.54 56.02,32.54 55.55,32.06 54.31,32.06 53.36,33.01 51.34,33.01 v50.56,33.03
  Bottom 0.203: C32.2 46.61,36.19 49.21,36.19 49.44,36.42 49.96,36.42 50.56,35.82 v50.56,33.03 50.33,32.8 50.33,32.72 49.96,32.35 49.44,32.35 49.21,32.58 48.5,32.58 47.16,31.23 47.16,31.1 45.13,29.07 45.13,21.33 42.34,18.54 37.5,18.54 37.43,18.47 37.43,18.46 37.06,18.09 36.46,18.09 35.83,18.72 34.84,18.72 32.21,21.35 R31.2
  other vias: 45.55,37.25 59.5,38.25 32.15,21.35 60.2,38.25 59.5,37.45 60.2,37.45 59.5,36.65 60.2,36.65 59.5,35.85 60.2,35.85 59.5,35.05 60.2,35.05 61.3,38.25 61.2,35.05 61.2,36.65 63,39.65 63.5,32.65 61.8,33.85 64.5,40.15 65.6,32.35 66.5,40.05 67,32.75 62.8,40.65 62.9,31.55
  pour Bottom (rank 3): 68.5,41.35 62.2,41.35 62.2,38.85 59.3,38.85 59.2,38.75 59.2,33.25 62.2,33.25 62.2,31.05 68.5,31.05
  pour Top (rank 3, no thermals): 68.5,41.35 59.2,41.35 59.2,34.45 60.5,34.45 61,33.95 61,32.35 60.3,31.65 59.2,31.65 59.2,31.15 59.3,31.05 68.5,31.05
PHASE-W  (via drill 0.35)  (1 unrouted)
  Top 0.203: U2.P$36 | C33.2 43.6,33.65 43.33,33.65 43.22,33.75 U2.P$36 | U$11.SH 59.82,25.93 60.38,25.93 60.56,25.75 60.56,24.57 60.05,24.06 58.95,24.06 58.58,24.44 55.92,24.44 55.55,24.06 50.74,24.06 v50.56,23.88 | v46.2,28.85 46.2,29.75 45.46,30.49 45.32,30.49 44.21,31.61 v43.89,31.61
  Bottom 0.203: v43.89,31.61 43.89,33.34 C33.2 | v50.56,23.88 49.8,24.64 49.8,25.84 50.33,26.37 50.33,26.9 49.96,27.27 47.78,27.27 v46.2,28.85 45.8,28.85 45.53,28.58 45.53,21.16 42.5,18.13 37.68,18.13 37.23,17.68 36.3,17.68 35.66,18.31 34.67,18.31 34.63,18.35 R36.2
  other vias: 43.9,33.35 59.6,30.15 32.15,18.35 60.3,30.15 59.6,29.35 60.3,29.35 59.6,28.55 60.3,28.55 59.6,27.75 60.3,27.75 59.6,26.95 60.3,26.95 61.5,30.15 61.6,28.25 61.6,26.25 63,30.15 63,28.55 63.1,27.35 64.5,30.15 64.5,28.55 66,28.55 66,30.15 66.5,27.35 67.6,21.05
  pour Top (rank 3, no thermals): 59.3,30.55 68.5,30.55 68.5,20.55 63.5,20.55 61,23.05 61,26.05 60.6,26.45 59.3,26.45
  pour Bottom (rank 3, no thermals): 68.5,30.55 59.3,30.55 59.3,24.75 63.5,20.55 68.5,20.55
PWMHI1
  Top 0.203: U2.P$17 32.78,35.75 32.27,35.24 28.29,35.24 28.24,35.28 27.5,35.28 27.27,35.51 27.27,35.81 26.9,36.19 26.49,36.19 25.83,36.85 25.83,38.81 25.4,39.25 25.4,41.21 J13.2 23.67,42.08 U1.29
PWMHI2
  Top 0.203: U2.P$19 32.93,34.75 32.56,34.38 32.38,34.38 32.33,34.42 27.95,34.42 27.91,34.47 27.01,34.47 26.56,34.92 26.24,34.92 26.01,35.15 26.01,36.1 25.43,36.68 25.43,38.64 J13.3 22.67,38.54 22.49,38.54 21.53,39.49 19.96,39.49 19.87,39.58 U1.24
PWMHI3
  Top 0.203: U2.P$21 33.08,33.75 32.89,33.56 32.04,33.56 31.99,33.61 27.61,33.61 27.57,33.66 26,33.66 25.6,34.06 25.6,35.93 J13.4 23.02,37.43 21.37,39.08 U1.23
PWMLO1  (via drill 0.35)
  Top 0.203: v26.64,35.55 26.64,35.42 27.18,34.88 28.07,34.88 28.12,34.83 32.44,34.83 32.86,35.25 U2.P$18 | v22,36.25 21.7,36.55 21.7,37.05 21.5,37.25 20.2,37.25 20.03,37.08 U1.19
  Bottom 0.203: v26.64,35.55 25.4,35.55 24.8,36.15 22.1,36.15 v22,36.25
PWMLO2  (via drill 0.35)
  Top 0.203: U1.18 19.42,36.51 19.78,36.51 19.96,36.34 19.96,36.05 21.13,34.88 21.47,34.88 v22,34.35 | U2.P$20 33,34.25 32.72,33.97 32.21,33.97 32.16,34.02 27.78,34.02 27.74,34.06 26.53,34.06 v26.3,34.29
  Bottom 0.203: v26.3,34.29 25.56,33.55 24.62,33.55 23.58,33.55 22.8,33.55 v22,34.35
PWMLO3
  Top 0.203: U1.17 21.88,33.55 23.58,33.55 24.62,33.55 24.89,33.55 24.9,33.55 25.2,33.25 27.4,33.25 27.45,33.2 31.83,33.2 31.88,33.16 33.06,33.16 33.1,33.2 33.94,33.2 U2.P$22
RESET  (via drill 0.35)
  Top 0.203: J1.10 7.01,36.46 7.45,36.9 v7.45,38.27 | U1.52 11.07,42.08 v11.1,42.05 | S1.P$2 17.8,49.3 R1.2 17.74,47.45 v16.9,47.45 | v9.8,49.15 v13,49.15
  Bottom 0.203: v7.45,38.27 7.56,38.39 | 7.56,38.39 9.02,39.84 10.03,39.84 10.57,39.31 10.57,38.99 10.94,38.62 11.46,38.62 11.83,38.99 11.83,39.51 11.46,39.88 11.14,39.88 10.5,40.52 10.5,41.45 v11.1,42.05 | v16.9,47.45 16.4,47.45 14.7,49.15 v13,49.15 | 7.56,38.39 6.7,39.25 6.7,46.75 9.1,49.15 v9.8,49.15
SHNT-V-HI  (via drill 0.35)
  Top 0.203: v35.1,19.35 R18.1
  Bottom 0.203: R4.SB 48.34,35.79 47.53,34.98 47.53,34.79 44.52,31.78 44.52,31.34 44.31,31.14 44.31,21.66 42,19.35 v35.1,19.35
  other vias: 49.7,35.79
SHNT-V-LO  (via drill 0.35)
  Top 0.203: v36.8,18.72 R19.1
  Bottom 0.203: R4.SA 48.34,32.99 46.75,31.4 46.75,31.27 44.72,29.24 44.72,21.5 42.17,18.94 37.03,18.94 v36.8,18.72
  other vias: 49.7,32.99
SHNT-W-HI  (via drill 0.35)
  Top 0.203: v38.5,17.5 R20.1
  Bottom 0.203: v38.5,17.5 38.73,17.72 42.67,17.72 45.94,20.99 45.94,25.49 47.09,26.64 R5.SB
  other vias: 49.7,26.64
SHNT-W-LO  (via drill 0.35)
  Top 0.203: v40.2,17.09 R21.1
  Bottom 0.203: R5.SA 49.7,24.16 49.39,24.47 49.39,24.94 48.1,26.23 47.25,26.23 46.34,25.32 46.34,20.82 42.84,17.32 40.4,17.32 40.2,17.12 v40.2,17.09
  other vias: 49.7,23.84
SL-V  (via drill 0.35)
  Top 0.203: U2.P$39 42.6,35.25 42.69,35.34 42.8,35.34 42.82,35.33 43.8,35.33 44.15,34.98 45.35,34.98 47.07,36.7 48.98,36.7 49.48,37.2 R4.B
  other vias: 54.3,38.25 55,38.25 54.3,37.45 55,37.45 54.3,36.65 55,36.65 54.3,35.85 55,35.85 54.3,35.05 55,35.05
  pour Top (no thermals): 49.4,38.15 52.6,38.15 53.8,39.35 53.9,39.35 55.3,39.35 55.4,39.25 55.4,34.05 55.4,33.95 55.3,33.85 49.4,33.85
  pour Bottom (rank 3, no thermals): 55.3,38.75 55.3,34.25 53.9,34.25 53.9,38.75
SL-W  (via drill 0.35)
  Top 0.203: U2.P$34 41.56,32.7 42.67,32.7 43.12,32.24 44.15,32.24 45.49,30.9 46.18,30.9 v47.17,29.91 | 50.26,28.48 50.67,28.48 | 51,28.48 50.67,28.48 | 50.67,28.48 50.45,28.7 | 50.45,28.7 50.3,28.85 | v48.88,29.55 48.88,29.17 49.35,28.7 50.45,28.7
  Bottom 0.203: v48.88,29.55 47.53,29.55 v47.17,29.91
  other vias: 55,30.25 54.3,30.25 55,29.45 54.3,29.45 55,28.65 54.3,28.65 55,27.85 54.3,27.85 55,27.05 54.3,27.05
  pour Top (no thermals): 55.3,30.75 54.2,30.75 52.4,28.95 47.5,28.95 47.5,25.55 49,24.05 54.4,24.05 55.3,24.95
  pour Bottom (rank 3, no thermals): 55.3,30.75 53.9,30.75 53.9,26.25 55.3,26.25
SPI_CSN
  Top 0.203: U1.41 14.6,44.96 14.73,45.09 14.73,45.61 14.36,45.98 13.67,45.98 13.5,46.15 13.5,47.13 J6.5
SPI_MISO
  Top 0.203: U1.44 13.1,44.88 13.06,44.92 13.06,45.44 12.38,46.12 12,46.12 11.43,46.69 J6.3
SPI_MOSI  (via drill 0.35)
  Top 0.203: U1.42 v14.1,45.35 | v14.4,48.45 14.43,48.42 J6.6
  Bottom 0.203: v14.1,45.35 14.1,48.15 v14.4,48.45
SPI_SCK
  Top 0.203: U1.43 13.6,44.96 13.47,45.09 13.47,45.61 12.43,46.65 J6.4
STL_ERROR  (via drill 0.35)
  Top 0.203: U1.62 10.28,37.01 9.69,37.01 8.27,35.59 v8.27,33.95
  Bottom 0.203: v8.27,33.95 8.27,30.07 R12.1
  other vias: 6.7,28.5
STL_TICKER  (via drill 0.35)
  Top 0.203: v11.2,37.55 10.38,37.55 U1.61
  Bottom 0.203: v11.2,37.55 11.2,36.58 10.3,35.68 8.74,35.68 7.64,34.58 7.64,31.19 R8.1
  other vias: 6.7,30.25
SWDCLK  (via drill 0.35)
  Top 0.203: J1.4 6.18,40.25 v7.34,40.25 | v11.2,39.25 10.87,39.58 U1.57
  Bottom 0.203: v11.2,39.25 10.2,40.25 v7.34,40.25
SWDIO
  Top 0.203: J1.2 6.95,41.54 8.09,40.39 8.09,39.84 8.3,39.63 9.33,39.63 9.88,39.08 U1.58
SWO
  Top 0.203: U1.59 9.54,38.58 9.51,38.55 9.51,38.24 9.33,38.06 8.27,38.06 8.09,38.24 8.09,38.57 7.66,39 J1.6
THERMISTOR
  Top 0.203: R14.1 R13.2
UP0RX  (via drill 0.35)
  Top 0.203: U1.14 17.6,35.85 v18.2,36.45 | v21.2,22.65 J5.P$2
  Bottom 0.203: v18.2,36.45 18.2,23.32 18.87,22.65 v21.2,22.65
UP0STLB
  Top 0.203: U1.60 9.99,38.08 9.75,37.84 9.75,37.65 7.64,35.53 7.64,33.69 8.3,33.02 R9.1
UP0STLR
  Top 0.203: U1.1 11.1,34.75 11.18,34.67 11.18,33.67 10.78,33.26 10.78,31.18 R7.1
UP0TX  (via drill 0.35)
  Top 0.203: U1.13 17.1,36.15 v16.9,36.35 | v17.2,18.85 v17.2,18.84 J5.P$5
  Bottom 0.203: v16.9,36.35 16.9,19.15 v17.2,18.85
UP1RX  (via drill 0.35)
  Top 0.203: U1.64 10.35,35.1 v10.3,35.05 | v17.1,8.95 17.15,8.91 J4.P$2
  Bottom 0.203: v10.3,35.05 10.3,15.75 v17.1,8.95
UP1STLB
  Top 0.203: U1.2 11.6,34.54 11.59,34.52 11.59,33.5 11.18,33.09 11.18,31.21 11.52,30.87 11.52,30.42 R16.1
UP1STLR
  Top 0.203: U1.3 12.1,34.46 11.99,34.36 11.99,33.33 11.59,32.92 11.59,31.38 12.01,30.96 12.04,30.96 R15.1
UP1TX  (via drill 0.35)
  Top 0.203: v16.8,5.15 16.85,5.1 J4.P$5 | U1.63 9.83,36.58 8.9,35.65 v8.9,34.95
  Bottom 0.203: v16.8,5.15 8.9,13.05 v8.9,34.95
V-U  (via drill 0.35)
  Top 0.203: R26.1 R27.2 30.1,25.85 29.4,25.15 27.51,25.15 C39.1 | D7.A 26.55,25.6 C39.1 | C39.1 26.7,25.75 25.16,25.75 J3.5 | U1.10 15.6,34.98 15.77,34.81 15.77,33.62 18.4,30.98 18.4,30.66 19.4,29.66 v19.4,29.45
  Bottom 0.203: v19.4,29.45 24.1,24.75 J3.5
V-V  (via drill 0.35)
  Top 0.203: R31.1 R32.2 29.9,22.85 29.2,22.14 27.51,22.14 C41.1 | D2.A 26.55,22.6 C41.1 | C41.1 24.8,22.85 J3.6 | U1.9 15.1,34.86 15.36,34.6 15.36,33.45 17.99,30.81 17.99,30.49 18.6,29.88 18.6,29.35 v19.4,28.55
  Bottom 0.203: v19.4,28.55 19.7,28.25 20.02,28.25 22.85,25.42 22.85,24.17 24.1,22.93 J3.6
V-VCC  (via drill 0.35)
  Top 0.203: R38.1 R39.2 30,16.85 29.3,16.14 27.41,16.14 26.75,16.8 | 26.75,16.8 C45.1 24.32,16.85 J3.8 | D5.A 26.55,16.6 26.75,16.8 | U1.5 13.1,34.77 13.49,34.39 13.49,31.67 13.91,31.26 15.54,31.26 18.36,28.44 18.36,27.8 19.14,27.02 19.17,27.02 v19.4,26.79
  Bottom 0.203: v19.4,26.79 20.33,26.79 22.04,25.08 22.04,23.84 22.39,23.49 22.39,18.78 J3.8
V-W  (via drill 0.35)
  Top 0.203: R36.1 R37.2 29.55,19.14 27.51,19.14 C43.1 | D3.A 26.8,18.6 C43.1 | C43.1 24.34,19.85 J3.7 | U1.6 13.6,34.85 13.9,34.55 13.9,31.84 14.07,31.66 15.71,31.66 18.77,28.61 18.77,28.29 v19.4,27.66 v19.4,27.65
  Bottom 0.203: v19.4,27.65 19.5,27.55 20.15,27.55 22.45,25.25 22.45,24.01 22.8,23.66 22.8,20.91 J3.7
VCC  (via drill 0.35)
  Top 0.203: R38.2 34,15.35
  other vias: 56.9,38.25 57.2,23.65 56.2,38.25 57.6,38.25 58.3,38.25 56.9,30.25 56.2,30.25 57.6,30.25 58.3,30.25 56.9,46.75 56.2,46.75 57.6,46.75 58.3,46.75 56.9,37.45 56.2,37.45 57.6,37.45 58.3,37.45 56.9,29.45 56.2,29.45 57.6,29.45 58.3,29.45 56.9,45.95 56.2,45.95 57.6,45.95 58.3,45.95 56.9,36.65 56.2,36.65 57.6,36.65 58.3,36.65 56.9,28.65 56.2,28.65 57.6,28.65 58.3,28.65 56.9,45.15 56.2,45.15 57.6,45.15 58.3,45.15 56.9,35.85 56.2,35.85 57.6,35.85 58.3,35.85 56.9,27.85 56.2,27.85 57.6,27.85 58.3,27.85 56.9,44.35 56.2,44.35 57.6,44.35 58.3,44.35 56.9,35.05 56.2,35.05 57.6,35.05 58.3,35.05 56.9,27.05 56.2,27.05 57.6,27.05 58.3,27.05 56.9,43.55 56.2,43.55 57.6,43.55 58.3,43.55 58.2,23.65 57.2,22.75 58.2,22.75 59.2,23.15 60,22.35 57.2,21.75 58.2,21.75 57.2,20.75 58.2,20.75 59.2,21.25 60.9,21.25 56.4,18.05 58.5,18.75 60.4,19.35 62.2,20.05 56.5,48.45 58,48.45 59.2,49.65 55,49.65 57.2,49.65 53.8,51.15 56.2,51.15 58.3,51.15 60.7,51.15 64.5,19.35 62.7,18.15 60.4,17.05 58.2,16.15 56.5,31.15 57.9,31.15 57.2,31.75 56.5,26.25 57.9,26.25 57.2,25.65 56.5,39.05 57.9,39.05 57.2,39.95 56.5,34.25 57.9,34.25 57.2,33.75 56.5,42.75 57.9,42.75 57.2,42.15 52.7,49.35 51.4,51.15
  pour Top (rank 5, no thermals): 25.75,52.25 25.75,27.75 33.75,27.75 33.75,13.25 54.5,13.25 55,12.75 55,0 68.5,0 68.5,52.25
  pour Bottom (rank 4): 55.4,48.05 55.3,18.55 63.7,8.25 68.5,8.25 68.5,20.35 63.4,20.35 59.2,24.55 59.1,30.85 59.3,31.05 61.9,31.05 61.9,32.85 61.8,32.95 59.3,32.95 59.1,33.15 59.1,38.95 59.3,39.15 61.9,39.15 61.9,41.35 59.3,41.35 59.1,41.55 59.1,48.15 62.5,51.55 62.5,52.25 49.7,52.25 49.8,48.05
VDDCORE
  Top 0.203: U1.53 9.08,41.58 | 9.08,41.58 C7.1 | C5.2 7.6,42.4 8.42,41.58 9.08,41.58

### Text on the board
tPlace: < no - go > | SPI | FAULT | U | HI1 | HI2 | HI3 | GND | V | 3V3 | I-V | W | I-W | V-U | V-V | V-W | UP0 | V-VCC | mkbldcdriver v0.4 | VCC | UP1 | GND
bPlace: since systems tend to leave unstable equilibria / they cannot often be in them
